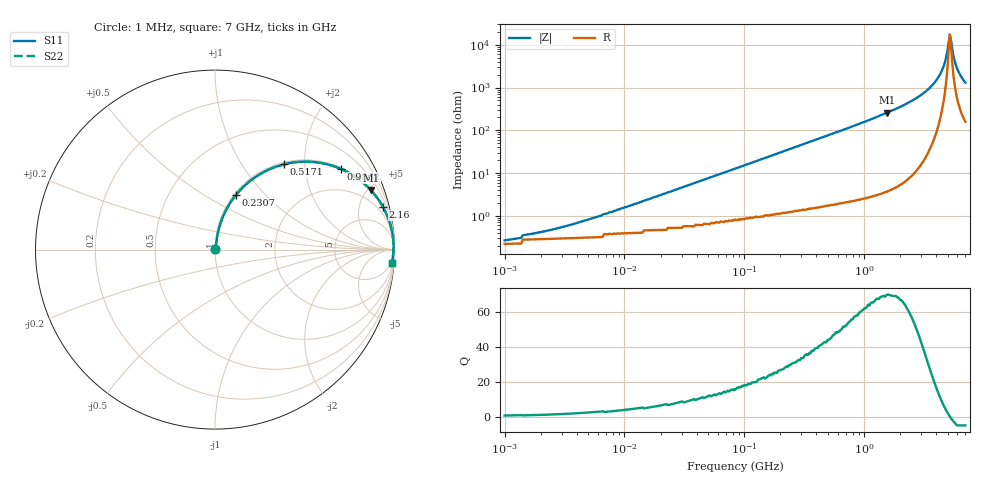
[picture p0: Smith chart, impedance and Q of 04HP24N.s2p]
# MHz S MA R 50
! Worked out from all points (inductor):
!   385 points, 1 MHz to 7 GHz, reference 50 ohm
!   read as one part in series: L = 24 nH near 6.473 MHz
!   highest Q = 69.7 at 1.564 GHz (marker M1), where L = 26.4 nH
!   self-resonance near 5.187 GHz
!   S11 on the Smith chart (normalised r, x): 1 MHz: 1.00, +0.00; 230.7 MHz: 1.02, +0.70; 517.1 MHz: 1.04, +1.57; 986.2 MHz: 1.05, +3.09; 2.16 GHz: 1.11, +7.87; 7 GHz: 4, -26
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1  0.002811 32.3  0.998 -0.1  0.998 -0.1  0.002811 32.3
2.044  0.004068 48.9  0.997 -0.2  0.997 -0.2  0.004068 48.9
4.374  0.007274 64.3  0.997 -0.4  0.997 -0.4  0.007274 64.3
19.575  0.03 79.3  0.995 -1.7  0.995 -1.7  0.03 79.3
85.617  0.127 79.2  0.984 -7.3  0.984 -7.3  0.127 79.2
230.745  0.326 69.0  0.934 -19.0  0.934 -19.0  0.326 69.0
365.931  0.48 59.8  0.865 -28.7  0.865 -28.7  0.48 59.8
517.128  0.612 51.0  0.777 -37.7  0.777 -37.7  0.612 51.0
986.21  0.833 32.7  0.54 -56.4  0.54 -56.4  0.833 32.7
1563.994  0.929 21.0  0.358 -68.2  0.358 -68.2  0.929 21.0
1637.803  0.935 19.9  0.341 -69.2  0.341 -69.2  0.935 19.9
2159.837  0.966 14.2  0.245 -74.9  0.245 -74.9  0.966 14.2
3196.293  0.988 7.3  0.128 -81.1  0.128 -81.1  0.988 7.3
4119.009  0.994 3.4  0.06 -82.6  0.06 -82.6  0.994 3.4
4730.122  0.995 1.4  0.025 -77.2  0.025 -77.2  0.995 1.4
4953.349  0.995 0.7  0.014 -66.7  0.014 -66.7  0.995 0.7
5187.11  0.994 0.1  0.005682 -9.2  0.005682 -9.2  0.994 0.1
5308.095  0.994 -0.3  0.00761 40.0  0.00761 40.0  0.994 -0.3
5558.598  0.994 -0.9  0.018 68.4  0.018 68.4  0.994 -0.9
5820.923  0.993 -1.6  0.029 75.0  0.029 75.0  0.993 -1.6
6095.627  0.992 -2.3  0.041 77.4  0.041 77.4  0.992 -2.3
7000  0.988 -4.3  0.076 78.7  0.076 78.7  0.988 -4.3
